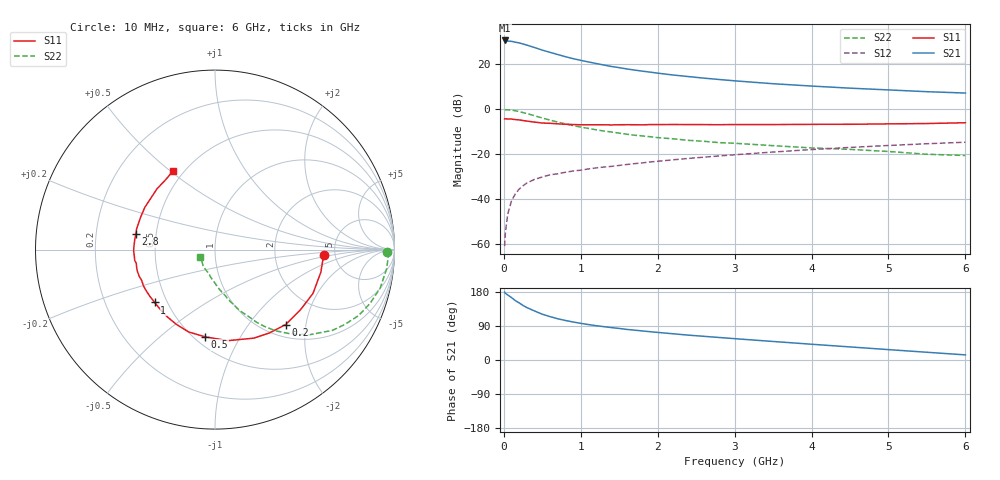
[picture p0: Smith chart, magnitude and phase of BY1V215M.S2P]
! SIEMENS Small Signal Semiconductors
! BFY420
! Si NPN RF SIEGET Grounded Emitter Transistor in MICRO-X
! VCE = 1.25 V  IC = 15 mA
! Common Emitter S-Parameters:  October  1996
# GHz  S  MA  R  50
!  f  S11  S21  S12  S22
! GHz  MAG  ANG  MAG  ANG  MAG  ANG  MAG  ANG
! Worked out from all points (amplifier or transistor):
!   36 points, 10 MHz to 6 GHz, reference 50 ohm
!   highest |S21| = 30.5 dB at 10 MHz (marker M1)
!   |S21| within 3 dB of that: start of sweep to 386.3 MHz
!   unconditionally stable (mu >= 1): 2.091 GHz to end of sweep
!   at 250 MHz: K = 0.25, MSG = 31.5 dB, |S12| = -34.1 dB
!   at 1.4 GHz: K = 0.87, MSG = 22.2 dB, |S12| = -25.5 dB
!   at 6 GHz: K = 1.09, MAG = 9.1 dB, |S12| = -14.7 dB
!   S11 on the Smith chart (normalised r, x): 10 MHz: 4.04, -0.36; 200 MHz: 1.24, -1.54; 500 MHz: 0.56, -0.72; 1 GHz: 0.43, -0.31; 2.8 GHz: 0.38, +0.08; 6 GHz: 0.44, +0.51
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0.01  0.6056 -2.7  33.33 179.0  0.0009 101.7  0.9611 -0.9
0.02  0.6042 -5.0  33.11 176.2  0.0018 97.4  0.9661 -2.2
0.05  0.603 -12.1  32.3 171.6  0.0046 83.8  0.9625 -6.3
0.1  0.5981 -24.1  31.82 164.7  0.0092 81.6  0.9454 -13.0
0.15  0.5824 -35.2  30.51 156.6  0.0131 74.9  0.9146 -19.1
0.2  0.5741 -46.7  29.36 150.6  0.0167 71.4  0.8803 -24.7
0.25  0.5544 -57.0  27.82 143.8  0.0198 66.7  0.8345 -30.0
0.3  0.5388 -66.3  26.23 138.3  0.0228 64.7  0.7944 -34.5
0.4  0.5123 -82.0  23.2 129.3  0.0275 59.0  0.7078 -42.1
0.5  0.4889 -96.6  20.32 120.8  0.0309 56.1  0.6311 -48.1
0.6  0.4817 -107.8  18.14 114.5  0.0346 54.6  0.5674 -53.0
0.7  0.4686 -117.4  16.24 108.9  0.0364 53.3  0.5138 -56.9
0.8  0.4595 -125.4  14.54 104.3  0.0394 51.6  0.4671 -60.2
1  0.447 -138.8  12.04 96.7  0.0439 50.9  0.3976 -65.0
1.1  0.4466 -144.6  11.11 93.5  0.0468 51.2  0.3707 -67.6
1.6  0.4491 -164.4  7.758 80.7  0.0587 51.1  0.2755 -76.2
2.2  0.4536 -179.3  5.695 69.2  0.0745 49.9  0.2181 -84.4
2.8  0.4491 169.0  4.525 59.4  0.0908 47.7  0.1795 -91.7
3.5  0.452 156.6  3.647 48.9  0.1109 43.6  0.1536 -99.5
4.5  0.4581 141.2  2.907 34.5  0.1405 35.7  0.1269 -112.0
5.5  0.4764 125.4  2.426 20.4  0.1695 26.7  0.099 -137.3
6  0.4959 118.2  2.265 13.5  0.1832 21.9  0.093 -155.1
